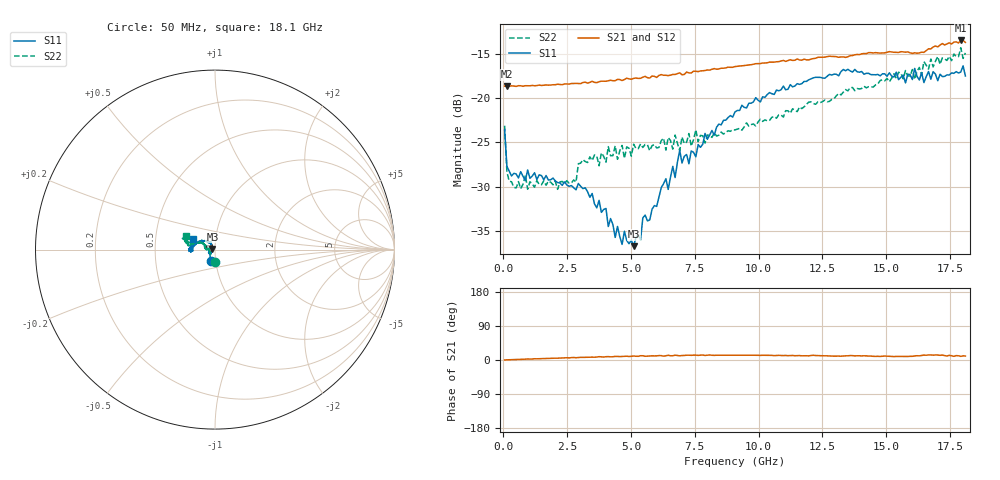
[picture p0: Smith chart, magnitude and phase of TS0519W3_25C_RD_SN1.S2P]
! Network Analyzer HP8720D.06.14 Serial No. US36140669
! 17 Jun 2005  09:20:23
! Frequency  S11  S21  S12  S22
# HZ  S  DB R 50
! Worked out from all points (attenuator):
!   201 points, 50 MHz to 18.1 GHz, reference 50 ohm
!   highest |S21| = -13.50 dB at 17.92 GHz (marker M1); lowest = -18.7 dB at 140.2 MHz (marker M2)
!   lowest |S11| = -36.7 dB at 5.104 GHz (marker M3), VSWR 1.03, Z = 48.6 + j0.324 ohm
!   |S11| at or under -10 dB: start of sweep to end of sweep
!   |S22| runs from -30.3 to -14.3 dB; largest |S21 - S12| = 0.0058
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5e7  -23.56 -111.2  -18.66 0.2  -18.61 0.4  -23.12 -89.3
1.4025e8  -27.71 -133.3  -18.69 0.4  -18.69 0.4  -28.34 -128.9
4.11e8  -28.51 -155.1  -18.64 1.1  -18.66 1.1  -30.08 -157.1
2.12575e9  -29.55 -146.7  -18.44 4.7  -18.49 4.8  -30.31 172.2
2.84775e9  -30.37 -136.8  -18.34 5.9  -18.36 6.2  -29.50 164.8
3.1185e9  -30.23 -145.4  -18.25 6.9  -18.30 6.8  -26.96 178.2
5.104e9  -36.73 166.8  -17.78 10.5  -17.71 10.2  -25.21 170.4
6.09675e9  -31.20 128.5  -17.45 11.7  -17.39 11.5  -25.58 169.7
6.3675e9  -29.11 127.4  -17.43 11.2  -17.45 11.7  -25.88 167.9
6.45775e9  -30.32 128.6  -17.47 12.6  -17.47 12.0  -24.46 166.7
6.63825e9  -27.71 126.5  -17.34 11.2  -17.38 11.5  -25.77 162.9
6.7285e9  -28.98 127.7  -17.34 12.7  -17.39 12.1  -24.18 164.0
6.909e9  -25.90 124.2  -17.15 11.1  -17.27 11.3  -25.93 159.5
7.27e9  -27.42 121.5  -17.16 12.8  -17.17 12.0  -24.01 161.7
7.36025e9  -25.98 120.2  -17.17 12.3  -17.15 12.8  -25.43 164.4
7.54075e9  -26.64 121.7  -16.98 12.9  -16.90 12.0  -23.60 164.1
7.90175e9  -24.00 131.5  -16.89 12.1  -16.88 12.4  -25.09 157.7
9.075e9  -21.57 143.5  -16.45 12.8  -16.45 12.7  -23.61 154.7
1.21435e10  -17.72 176.3  -15.54 12.5  -15.54 12.2  -20.62 154.5
1.512175e10  -17.15 -177.8  -14.76 9.9  -14.75 10.1  -18.17 165.0
1.79195e10  -17.06 153.5  -13.50 9.6  -13.28 10.1  -14.32 161.1
1.81e10  -17.51 154.4  -13.71 10.5  -13.72 9.0  -14.91 155.5
